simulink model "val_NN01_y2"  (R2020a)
settings: Solver=ode45  StartTime=0.0  StopTime=100  RelTol=1e-3  EnableMultiTasking=on
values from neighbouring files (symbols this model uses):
  Ts = 0.05    [init_model.m]
libraries: neural x26

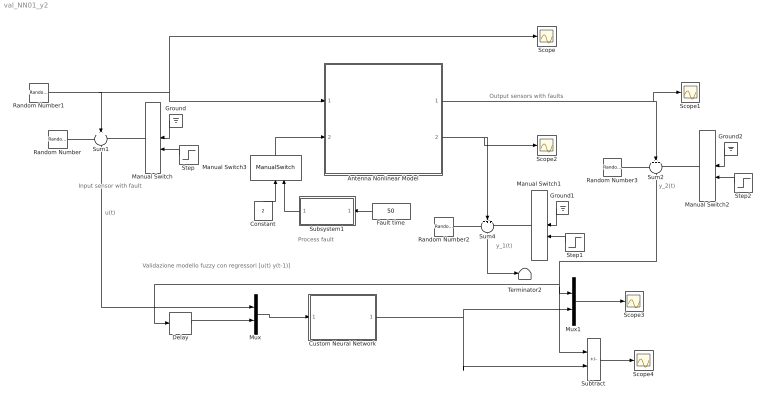
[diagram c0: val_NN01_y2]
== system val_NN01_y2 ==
  note: Validazione modello fuzzy con regressori [u(t) y(t-1)]
  note: u(t)
  note: Output sensors with faults
  note: Process fault
  note: Input sensor with fault
  note: y_1(t)
  note: y_2(t)
  Antenna Nonlinear Model : Subsystem
  Constant : Constant  Value=2
  Custom Neural Network : Subsystem
      mask help: Custom Neural Network
  Delay : Delay  DelayLength=1  SampleTime=Ts
  Fault time : Constant  Value=50
  Ground : Ground
  Ground1 : Ground
  Ground2 : Ground
  Manual Switch : ManualSwitch
  Manual Switch1 : ManualSwitch  CurrentSetting=0
  Manual Switch2 : ManualSwitch
  Manual Switch3 : ManualSwitch
  Mux : Mux  Inputs=2
  Mux1 : Mux  Inputs=2
  Random Number : RandomNumber  Variance=0.0001  Seed=1  SampleTime=Ts
  Random Number1 : RandomNumber  Variance=0.1  SampleTime=10
  Random Number2 : RandomNumber  Variance=0.00001  Seed=2  SampleTime=Ts
  Random Number3 : RandomNumber  Variance=0.00001  Seed=3  SampleTime=Ts
  Scope{,1..4} (5 alike) : Scope
  Step : Step  Time=50  SampleTime=0
  Step1 : Step  Time=50  SampleTime=0
  Step2 : Step  Time=50  SampleTime=0
  Subsystem1 : Subsystem
  Subtract : Sum  Inputs=+-
  Sum1 : Sum  Inputs=+++  SaturateOnIntegerOverflow=on
  Sum2 : Sum  Inputs=+++  SaturateOnIntegerOverflow=on
  Sum4 : Sum  Inputs=+++  SaturateOnIntegerOverflow=on
  Terminator2 : Terminator
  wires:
  Random Number1/1 -> Scope/1, Antenna Nonlinear Model/1(force), Sum1/2
  Random Number/1 -> Sum1/1
  Manual Switch/1 -> Sum1/3
  Sum1/1 -> Mux/1
  Ground/1 -> Manual Switch/1
  Step/1 -> Manual Switch/2
  Random Number2/1 -> Sum4/1
  Ground1/1 -> Manual Switch1/1
  Manual Switch1/1 -> Sum4/3
  Step1/1 -> Manual Switch1/2
  Antenna Nonlinear Model/2(velocity) -> Sum4/2, Scope2/1
  Random Number3/1 -> Sum2/1
  Ground2/1 -> Manual Switch2/1
  Manual Switch2/1 -> Sum2/3
  Step2/1 -> Manual Switch2/2
  Antenna Nonlinear Model/1(angle) -> Sum2/2, Scope1/1
  Sum2/1 -> Subtract/1, Mux1/1, Delay/1
  Fault time/1 -> Subsystem1/1(Fault time)
  Subsystem1/1(Fault) -> Manual Switch3/2
  Manual Switch3/1 -> Antenna Nonlinear Model/2(drag)
  Constant/1 -> Manual Switch3/1
  Delay/1 -> Mux/2
  Mux/1 -> Custom Neural Network/1(Input)
  Custom Neural Network/1(Output) -> Subtract/2, Mux1/2
  Mux1/1 -> Scope3/1
  Subtract/1 -> Scope4/1
  Sum4/1 -> Terminator2/1

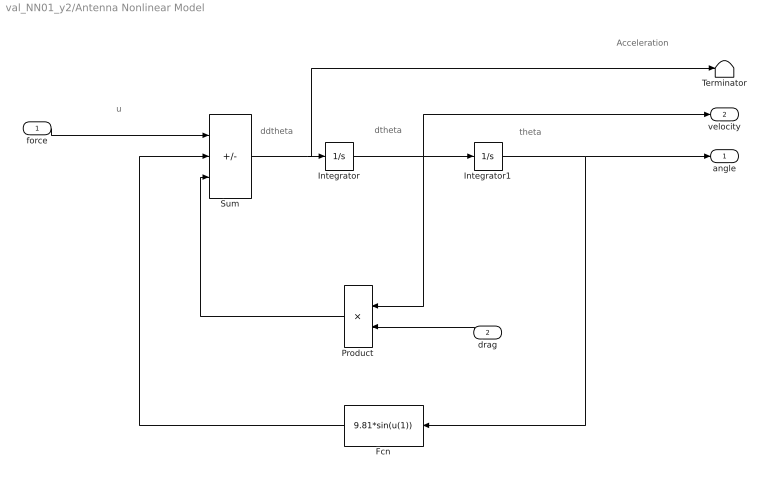
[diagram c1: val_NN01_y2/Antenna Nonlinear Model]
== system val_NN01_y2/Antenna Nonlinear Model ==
  note: Acceleration
  note: ddtheta
  note: dtheta
  note: theta
  note: u
  force : Inport
  drag : Inport  Port=2
  Fcn : Fcn  Expr=9.81*sin(u(1))
  Integrator : Integrator
  Integrator1 : Integrator  InitialCondition=(pi/180)*90
  Product : Product
  Sum : Sum  Inputs=+--  SaturateOnIntegerOverflow=on
  Terminator : Terminator
  angle : Outport
  velocity : Outport  Port=2
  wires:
  Sum/1 -> Terminator/1, Integrator/1
  Integrator/1 -> Product/1, Integrator1/1, velocity/1
  Integrator1/1 -> angle/1, Fcn/1
  Fcn/1 -> Sum/2
  Product/1 -> Sum/3
  force/1 -> Sum/1
  drag/1 -> Product/2

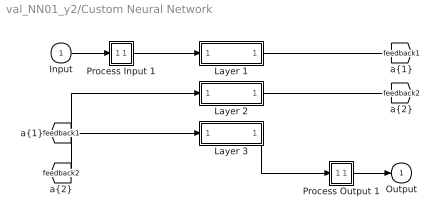
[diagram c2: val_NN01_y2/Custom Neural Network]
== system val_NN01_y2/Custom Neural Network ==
  Input : Inport  PortDimensions=3  SampleTime=0.05
  Layer 1 : Subsystem
  Layer 2 : Subsystem
  Layer 3 : Subsystem
  Process Input 1 : Subsystem
  Process Output 1 : Subsystem
  Output : Outport  InitialOutput=0
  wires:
  Input/1 -> Process Input 1/1(x)
  Process Output 1/1(y) -> Output/1
  Process Input 1/1(p) -> Layer 1/1("p{1}")
  Layer 1/1("a{1}") -> [feedback1]
  [feedback1] -> Layer 2/1("a{1} ")
  Layer 2/1("a{2}") -> [feedback2]
  [feedback2] -> Layer 3/1("a{2} ")
  Layer 3/1("a{3}") -> Process Output 1/1(a)

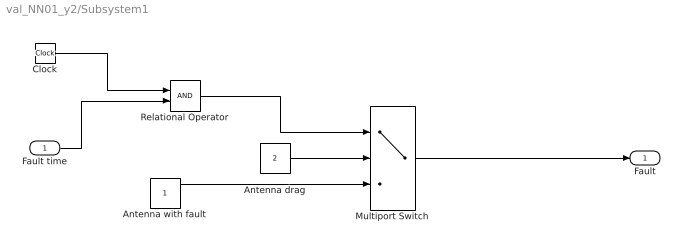
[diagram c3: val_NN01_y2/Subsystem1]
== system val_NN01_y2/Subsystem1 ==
  Fault time : Inport
  Antenna drag : Constant  Value=2
  Antenna with fault : Constant
  Clock : Clock
  Multiport Switch : MultiPortSwitch  DataPortOrder=Zero-based contiguous  Inputs=2  zeroidx=on
  Relational Operator : RelationalOperator  OutDataTypeStr=boolean  RndMeth=Simplest
  Fault : Outport
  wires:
  Clock/1 -> Relational Operator/1
  Fault time/1 -> Relational Operator/2
  Antenna drag/1 -> Multiport Switch/2
  Relational Operator/1 -> Multiport Switch/1
  Multiport Switch/1 -> Fault/1
  Antenna with fault/1 -> Multiport Switch/3

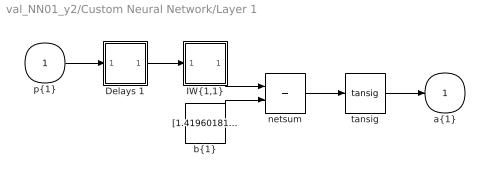
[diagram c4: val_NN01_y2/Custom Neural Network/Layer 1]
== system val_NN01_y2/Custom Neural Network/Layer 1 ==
  "p{1}" : Inport  PortDimensions=3  SampleTime=0.05
  Delays 1 : Subsystem
  "IW{1,1}" : Subsystem
  "b{1}" : Constant  Value=[1.419601812874873747460924278129823505878448486328125;0.54877143539052053444748935362440533936023712158203125;0.67746609781261735161450587838771753013134002685546875;-1.138497051044549568388219995540566742420196533203125;-0.43094892760474456938624143731431104242801666259765625;-2.384880970353273621498146894737146794795989990234375;2.6501087196827644021368541871197521686553955078125]
  netsum : Sum  Inputs=2  InputSameDT=on  SaturateOnIntegerOverflow=on
  tansig : neural/Transfer Functions/tansig
  "a{1}" : Outport  InitialOutput=[0;0;0;0;0;0;0]
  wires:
  "p{1}"/1 -> Delays 1/1("p{1}")
  Delays 1/1("pd{1,1}") -> "IW{1,1}"/1("pd{1,1}")
  "IW{1,1}"/1("iz{1,1}") -> netsum/1
  "b{1}"/1 -> netsum/2
  netsum/1 -> tansig/1
  tansig/1 -> "a{1}"/1

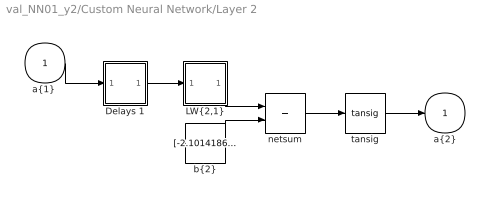
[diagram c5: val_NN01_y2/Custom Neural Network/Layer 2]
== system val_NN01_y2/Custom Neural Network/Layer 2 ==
  "a{1} " : Inport  PortDimensions=7  SampleTime=0.05
  Delays 1 : Subsystem
  "LW{2,1}" : Subsystem
  "b{2}" : Constant  Value=[-2.101418643619037407432870168122462928295135498046875;1.88791458750977625413725036196410655975341796875;-1.3493867656540035060430682278820313513278961181640625;1.368986560620593539994160892092622816562652587890625;-0.928828488295339038671727394103072583675384521484375;0.81898708879499027002424327292828820645809173583984375;0.273537385610062411256393488656613044440746307373046875;-0.0503570363679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
  netsum : Sum  Inputs=2  InputSameDT=on  SaturateOnIntegerOverflow=on
  tansig : neural/Transfer Functions/tansig
  "a{2}" : Outport  InitialOutput=[0;0;0;0;0;0;0;0;0;0;0;0;0;0;0]
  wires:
  "a{1} "/1 -> Delays 1/1("p{2}")
  Delays 1/1("pd{2,1}") -> "LW{2,1}"/1("ad{2,1}")
  "LW{2,1}"/1("lz{2,1}") -> netsum/1
  "b{2}"/1 -> netsum/2
  netsum/1 -> tansig/1
  tansig/1 -> "a{2}"/1

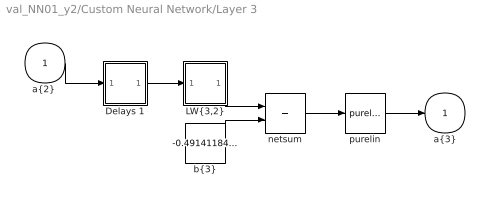
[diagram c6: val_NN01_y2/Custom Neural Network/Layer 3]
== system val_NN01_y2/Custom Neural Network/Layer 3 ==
  "a{2} " : Inport  PortDimensions=15  SampleTime=0.05
  Delays 1 : Subsystem
  "LW{3,2}" : Subsystem
  "b{3}" : Constant  Value=-0.491411847697218073793834491880261339247226715087890625
  netsum : Sum  Inputs=2  InputSameDT=on  SaturateOnIntegerOverflow=on
  purelin : neural/Transfer Functions/purelin
  "a{3}" : Outport  InitialOutput=0
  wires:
  "a{2} "/1 -> Delays 1/1("p{3}")
  Delays 1/1("pd{3,2}") -> "LW{3,2}"/1("ad{3,2}")
  "LW{3,2}"/1("lz{3,2}") -> netsum/1
  "b{3}"/1 -> netsum/2
  netsum/1 -> purelin/1
  purelin/1 -> "a{3}"/1

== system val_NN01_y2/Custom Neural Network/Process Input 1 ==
  x : Inport  PortDimensions=3  SampleTime=0.05
  p : Outport  PortDimensions=3  SampleTime=0.05
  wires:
  x/1 -> p/1

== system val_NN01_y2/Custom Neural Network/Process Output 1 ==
  a : Inport  PortDimensions=1  SampleTime=0.05
  y : Outport  PortDimensions=1  SampleTime=0.05
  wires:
  a/1 -> y/1

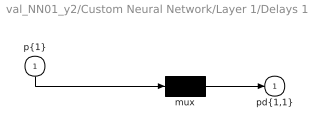
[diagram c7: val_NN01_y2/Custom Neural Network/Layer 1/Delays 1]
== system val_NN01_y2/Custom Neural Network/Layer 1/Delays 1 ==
  "p{1}" : Inport  PortDimensions=3  SampleTime=0.05
  mux : Mux  Inputs=1
  "pd{1,1}" : Outport
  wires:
  "p{1}"/1 -> mux/1
  mux/1 -> "pd{1,1}"/1

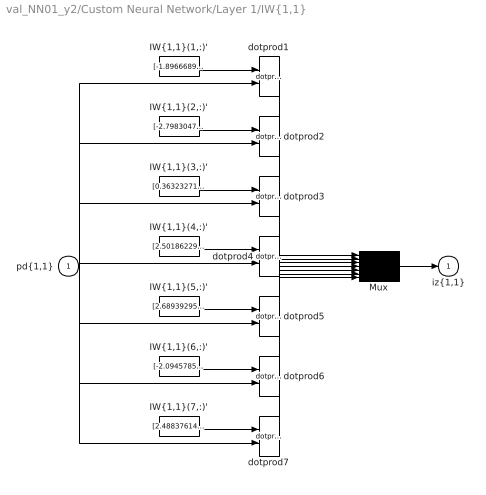
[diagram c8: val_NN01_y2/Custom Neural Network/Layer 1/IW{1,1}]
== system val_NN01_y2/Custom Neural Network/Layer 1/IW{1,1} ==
  "pd{1,1}" : Inport  PortDimensions=3  SampleTime=0.05
  "IW{1,1}(1,:)'" : Constant  Value=[-1.89666896675382901094053522683680057525634765625;2.38464493585232784056415766826830804347991943359375;1.6683249040604242185992234226432628929615020751953125]
  "IW{1,1}(2,:)'" : Constant  Value=[-2.79830477672292321500435718917287886142730712890625;-0.023799812840716132178453534606887842528522014617919921875;1.367477467874178120865735763800330460071563720703125]
  "IW{1,1}(3,:)'" : Constant  Value=[0.36323271241664445430075147669413127005100250244140625;1.585725010154640290949146219645626842975616455078125;-2.268472519700562628486295579932630062103271484375]
  "IW{1,1}(4,:)'" : Constant  Value=[2.5018622987315524142104550264775753021240234375;-1.813005103116014371522624060162343084812164306640625;1.05703421316772594451549593941308557987213134765625]
  "IW{1,1}(5,:)'" : Constant  Value=[2.689392955095101900298004693468101322650909423828125;-0.61918722817194737917390057191369123756885528564453125;1.7945478112426236361187648071791045367717742919921875]
  "IW{1,1}(6,:)'" : Constant  Value=[-2.094578517903359138330188216059468686580657958984375;2.566364336404209911535190258291549980640411376953125;1.0344427760634378188342452631331980228424072265625]
  "IW{1,1}(7,:)'" : Constant  Value=[2.488376140601343156077973617357201874256134033203125;1.54440643703103841488655234570614993572235107421875;1.1664770148498602164721660301438532769680023193359375]
  Mux : Mux  Inputs=7
  dotprod{1..7} (7 alike) : neural/Weight Functions/dotprod
  "iz{1,1}" : Outport
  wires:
  "IW{1,1}(1,:)'"/1 -> dotprod1/1
  "pd{1,1}"/1 -> dotprod1/2, dotprod2/2, dotprod3/2, dotprod4/2, dotprod5/2, dotprod6/2, dotprod7/2
  dotprod1/1 -> Mux/1
  "IW{1,1}(2,:)'"/1 -> dotprod2/1
  dotprod2/1 -> Mux/2
  "IW{1,1}(3,:)'"/1 -> dotprod3/1
  dotprod3/1 -> Mux/3
  "IW{1,1}(4,:)'"/1 -> dotprod4/1
  dotprod4/1 -> Mux/4
  "IW{1,1}(5,:)'"/1 -> dotprod5/1
  dotprod5/1 -> Mux/5
  "IW{1,1}(6,:)'"/1 -> dotprod6/1
  dotprod6/1 -> Mux/6
  "IW{1,1}(7,:)'"/1 -> dotprod7/1
  dotprod7/1 -> Mux/7
  Mux/1 -> "iz{1,1}"/1

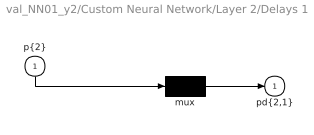
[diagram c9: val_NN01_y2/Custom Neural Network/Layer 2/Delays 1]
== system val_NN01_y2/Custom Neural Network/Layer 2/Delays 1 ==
  "p{2}" : Inport  PortDimensions=7  SampleTime=0.05
  mux : Mux  Inputs=1
  "pd{2,1}" : Outport
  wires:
  "p{2}"/1 -> mux/1
  mux/1 -> "pd{2,1}"/1

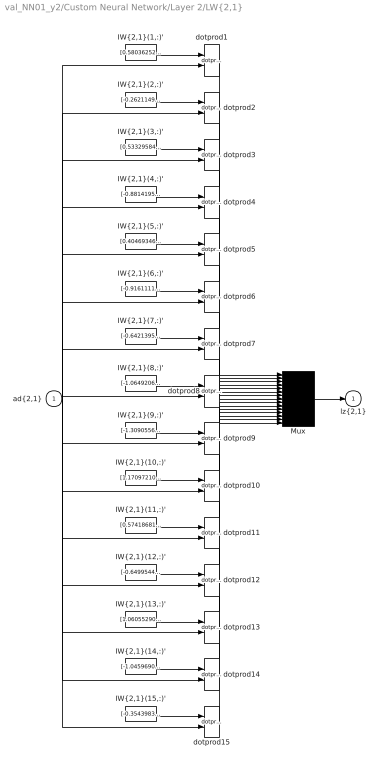
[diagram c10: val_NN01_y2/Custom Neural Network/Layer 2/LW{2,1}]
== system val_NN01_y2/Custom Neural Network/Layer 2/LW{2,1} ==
  "ad{2,1}" : Inport  PortDimensions=7  SampleTime=0.05
  "IW{2,1}(1,:)'" : Constant  Value=[0.5803625252357391683943887983332388103008270263671875;-0.133705302459637354051125157639035023748874664306640625;1.0806182154570571629648156886105425655841827392578125;-0.64937722682725596001773737953044474124908447265625;0.643886755822188572295772246434353291988372802734375;1.0399304006244605158570948333363048732280731201171875;0.04130813296219233710093732270252075977623462677001953125]
  "IW{2,1}(10,:)'" : Constant  Value=[1.170972106494776898699683442828245460987091064453125;-0.31872604913538105098069763698731549084186553955078125;0.8260295989341972511255107747274450957775115966796875;-0.1057765030127619521049808781754109077155590057373046875;-0.61593150776778637922603820697986520826816558837890625;-0.258436307205640869444351892525446601212024688720703125;1.1663071807726321793552415329031646251678466796875]
  "IW{2,1}(11,:)'" : Constant  Value=[0.57418681034918994665616764905280433595180511474609375;0.418637267311688432425142991633038036525249481201171875;0.279588602149626608284194162479252554476261138916015625;0.9410793609815486515657312338589690625667572021484375;0.274137400987252199957566745069925673305988311767578125;-1.0772091389571887276588313397951424121856689453125;-1.2025005515861051375026136156520806252956390380859375]
  "IW{2,1}(12,:)'" : Constant  Value=[-0.649954430278405492771298668230883777141571044921875;0.5739997492147701496634226714377291500568389892578125;-1.4091371295329844226529303341521881520748138427734375;0.4290792297889216566630921079195104539394378662109375;-0.090588165354822003383361561645870096981525421142578125;-0.85708506647996840488445968730957247316837310791015625;-0.379777327049689084059735932896728627383708953857421875]
  "IW{2,1}(13,:)'" : Constant  Value=[1.0605529022493549451411354311858303844928741455078125;-0.706726847331670793295188559568487107753753662109375;-0.6925027407876760410232463982538320124149322509765625;0.111513593105729225118949443640303798019886016845703125;-1.059091408542044643326107689063064754009246826171875;0.896253818909210853149716058396734297275543212890625;-0.434662294849831265519668477281811647117137908935546875]
  "IW{2,1}(14,:)'" : Constant  Value=[-1.045969004726185147546857479028403759002685546875;-0.989800953922295168041500801336951553821563720703125;-0.467033260286264961802515927047352306544780731201171875;0.9173359365680473498372293761349283158779144287109375;-0.277439251392562702402955210345680825412273406982421875;-1.0131560680427897924715807675966061651706695556640625;0.83481169703041724350356389550142921507358551025390625]
  "IW{2,1}(15,:)'" : Constant  Value=[-0.354398325297973049163857695020851679146289825439453125;-0.1683715305519686011859192831252585165202617645263671875;0.9901830089882306396020794636569917201995849609375;-0.5614947876994289543972627143375575542449951171875;-0.95256442068323610161684200647869147360324859619140625;1.024322616548112296896988482330925762653350830078125;-0.38396301693538881227851788935367949306964874267578125]
  "IW{2,1}(2,:)'" : Constant  Value=[-0.2621149401286058111537613513064570724964141845703125;0.8194121044772673112532856976031325757503509521484375;-0.46202708938246483949541243418934755027294158935546875;0.74377283349605483042665809989557601511478424072265625;0.5908072763607992161638549077906645834445953369140625;-0.71249568056545020677816637544310651719570159912109375;1.1791041866976568197600272469571791589260101318359375]
  "IW{2,1}(3,:)'" : Constant  Value=[0.53329584316601474913710490000084973871707916259765625;1.0772225679138383025446046303841285407543182373046875;0.1309398727908392123797653994188294745981693267822265625;-0.92005757445224867208111163563444279134273529052734375;-0.428207794053561630054360875874408520758152008056640625;-0.10614368315482093640955696400851593352854251861572265625;-1.330075806617494915684574152692221105098724365234375]
  "IW{2,1}(4,:)'" : Constant  Value=[-0.88141957883815968965990350625361315906047821044921875;-0.5825232039420760177250713240937329828739166259765625;-0.4944220259939762218692749229376204311847686767578125;0.894824693767890977369461324997246265411376953125;0.02166406946108311026844006619285210035741329193115234375;-1.0715258829539318075063647484057582914829254150390625;0.06918314059348802669280331656409543938934803009033203125]
  "IW{2,1}(5,:)'" : Constant  Value=[0.404693463800271491237481313874013721942901611328125;-0.2239498980349179102500301041800412349402904510498046875;0.98993775321197963190655855214572511613368988037109375;-0.336638094686156852386460514026111923158168792724609375;-1.019457368380464412638275462086312472820281982421875;0.310159663669201279834197748641599901020526885986328125;-0.90230302225502445612193014312651939690113067626953125]
  "IW{2,1}(6,:)'" : Constant  Value=[-0.91611117791475249472199493538937531411647796630859375;0.406313979341823172664049934610375203192234039306640625;-0.967737446884622709575296539696864783763885498046875;-0.4182833088851596325952186816721223294734954833984375;-0.76801256340283818868641674271202646195888519287109375;-0.62045561156288953075232939227134920656681060791015625;1.320006129549728957073284618672914803028106689453125]
  "IW{2,1}(7,:)'" : Constant  Value=[-0.64213958443884477933494281387538649141788482666015625;0.48677140740166280341583160407026298344135284423828125;0.06376429552227935726449459252762608230113983154296875;-0.87291735611115084392253038458875380456447601318359375;0.0279227761869431934105278969582286663353443145751953125;0.5934887370860091326818519519292749464511871337890625;-1.64354658852062840423968737013638019561767578125]
  "IW{2,1}(8,:)'" : Constant  Value=[-1.06492069087280327721600770018994808197021484375;0.29854850741403404779106267596944235265254974365234375;0.69643073880333028480293933171196840703487396240234375;0.614516886061886591363645493402145802974700927734375;1.07358571787202894398660646402277052402496337890625;0.85345539647470591848588128414121456444263458251953125;0.881619581805048735390073488815687596797943115234375]
  "IW{2,1}(9,:)'" : Constant  Value=[-1.3090556489412363827540275451610796153545379638671875;0.4387836328915935002470405379426665604114532470703125;0.833751029391784914679419671301729977130889892578125;-0.24275688151098406830641351916710846126079559326171875;1.0305834024823068428844408117583952844142913818359375;0.336362570438061114774797033533104695379734039306640625;0.58083131113498531750138909046654589474201202392578125]
  Mux : Mux  Inputs=15
  dotprod{1..15} (15 alike) : neural/Weight Functions/dotprod
  "lz{2,1}" : Outport
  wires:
  "IW{2,1}(1,:)'"/1 -> dotprod1/1
  "ad{2,1}"/1 -> dotprod1/2, dotprod2/2, dotprod3/2, dotprod4/2, dotprod5/2, dotprod6/2, dotprod7/2, dotprod8/2, dotprod9/2, dotprod10/2, dotprod11/2, dotprod12/2, dotprod13/2, dotprod14/2, dotprod15/2
  dotprod1/1 -> Mux/1
  "IW{2,1}(2,:)'"/1 -> dotprod2/1
  dotprod2/1 -> Mux/2
  "IW{2,1}(3,:)'"/1 -> dotprod3/1
  dotprod3/1 -> Mux/3
  "IW{2,1}(4,:)'"/1 -> dotprod4/1
  dotprod4/1 -> Mux/4
  "IW{2,1}(5,:)'"/1 -> dotprod5/1
  dotprod5/1 -> Mux/5
  "IW{2,1}(6,:)'"/1 -> dotprod6/1
  dotprod6/1 -> Mux/6
  "IW{2,1}(7,:)'"/1 -> dotprod7/1
  dotprod7/1 -> Mux/7
  "IW{2,1}(8,:)'"/1 -> dotprod8/1
  dotprod8/1 -> Mux/8
  "IW{2,1}(9,:)'"/1 -> dotprod9/1
  dotprod9/1 -> Mux/9
  "IW{2,1}(10,:)'"/1 -> dotprod10/1
  dotprod10/1 -> Mux/10
  "IW{2,1}(11,:)'"/1 -> dotprod11/1
  dotprod11/1 -> Mux/11
  "IW{2,1}(12,:)'"/1 -> dotprod12/1
  dotprod12/1 -> Mux/12
  "IW{2,1}(13,:)'"/1 -> dotprod13/1
  dotprod13/1 -> Mux/13
  "IW{2,1}(14,:)'"/1 -> dotprod14/1
  dotprod14/1 -> Mux/14
  "IW{2,1}(15,:)'"/1 -> dotprod15/1
  dotprod15/1 -> Mux/15
  Mux/1 -> "lz{2,1}"/1

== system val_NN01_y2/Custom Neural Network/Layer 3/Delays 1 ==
  "p{3}" : Inport  PortDimensions=15  SampleTime=0.05
  mux : Mux  Inputs=1
  "pd{3,2}" : Outport
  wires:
  "p{3}"/1 -> mux/1
  mux/1 -> "pd{3,2}"/1

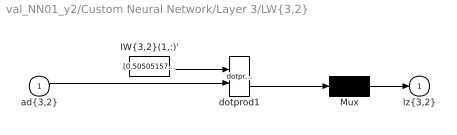
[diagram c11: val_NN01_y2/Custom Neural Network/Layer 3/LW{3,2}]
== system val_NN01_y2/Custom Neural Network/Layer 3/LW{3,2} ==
  "ad{3,2}" : Inport  PortDimensions=15  SampleTime=0.05
  "IW{3,2}(1,:)'" : Constant  Value=[0.50505157774393849567928782562375999987125396728515625;-0.40690011357376543177366556847118772566318511962890625;-0.211803799603253739558539336940157227218151092529296875;-0.47791404271533466374677345811505801975727081298828125;-0.29539158797351661167596148516167886555194854736328125;0.577382163373490353563965982175432145595550537109375;-0.007953014722455891555297213812991685699671506881713867187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
  Mux : Mux  Inputs=1
  dotprod1 : neural/Weight Functions/dotprod
  "lz{3,2}" : Outport
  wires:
  "IW{3,2}(1,:)'"/1 -> dotprod1/1
  "ad{3,2}"/1 -> dotprod1/2
  dotprod1/1 -> Mux/1
  Mux/1 -> "lz{3,2}"/1
